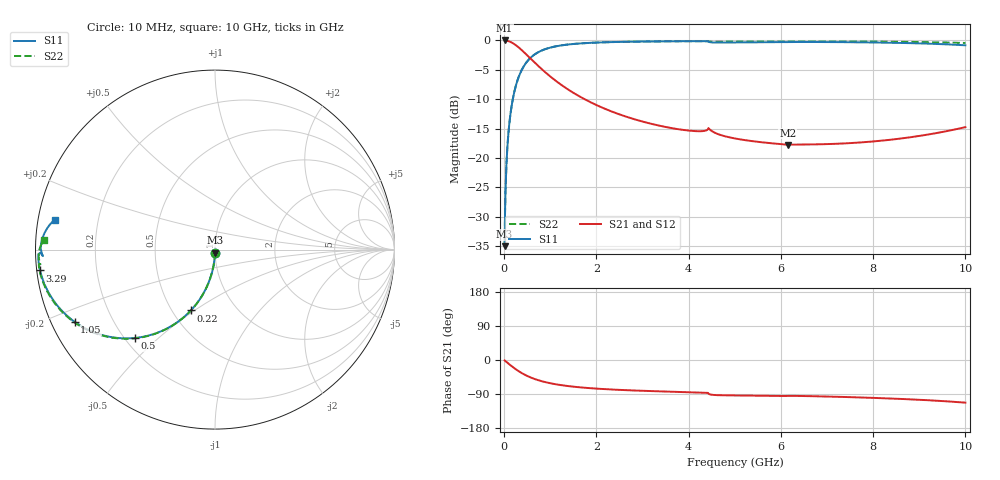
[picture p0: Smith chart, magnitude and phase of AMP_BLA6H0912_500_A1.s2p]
! Created Mon Feb  1 16:19:20 2010
# hz S ma R 50
! 2 Port Network Data from SP1.SP block
! freq  magS11  angS11  magS21  angS21  magS12  angS12  magS22  angS22
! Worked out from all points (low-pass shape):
!   1000 points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, 10 MHz to 10 GHz, reference 50 ohm
!   highest |S21| = 0.00 dB at 10 MHz (marker M1); lowest = -17.7 dB at 6.15 GHz (marker M2)
!   |S21| within 3 dB of the highest: start of sweep to 562.3 MHz
!   lowest |S11| = -35.0 dB at 10 MHz (marker M3), VSWR 1.04, Z = 49.9 - j1.78 ohm
!   |S11| at or under -10 dB: start of sweep to 187.2 MHz
!   |S22| runs from -35.0 to -0.1 dB; largest |S21 - S12| = 0
!   S11 on the Smith chart (normalised r, x): 10 MHz: 1.00, -0.04; 220 MHz: 0.62, -0.48; 500 MHz: 0.24, -0.42; 1.05 GHz: 0.07, -0.24; 3.29 GHz: 0.01, -0.06; 10 GHz: 0.05, +0.09
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1e7  0.01782 -91.0  0.9998 -1.0  0.9998 -1.0  0.01782 -91.0
4e7  0.07112 -94.1  0.9975 -4.1  0.9975 -4.1  0.07112 -94.1
7e7  0.1238 -97.2  0.9923 -7.2  0.9923 -7.2  0.1238 -97.2
1e8  0.1755 -100.2  0.9845 -10.2  0.9845 -10.2  0.1755 -100.2
1.5e8  0.2582 -105.1  0.9661 -15.1  0.9661 -15.1  0.2582 -105.1
2.2e8  0.3649 -111.6  0.9311 -21.6  0.9311 -21.6  0.3649 -111.6
3.4e8  0.5177 -121.6  0.8556 -31.5  0.8556 -31.5  0.5177 -121.4
5e8  0.6641 -132.2  0.7477 -42.1  0.7477 -42.1  0.6641 -132.0
7.5e8  0.7986 -143.8  0.6018 -53.7  0.6018 -53.7  0.7986 -143.5
1.05e9  0.8792 -152.7  0.4764 -62.5  0.4764 -62.5  0.8792 -152.3
1.33e9  0.9183 -158.2  0.3959 -67.9  0.3959 -67.9  0.9183 -157.6
1.68e9  0.9451 -162.9  0.3267 -72.5  0.3267 -72.5  0.9451 -162.2
2.43e9  0.9706 -169.0  0.2407 -78.5  0.2407 -78.5  0.9706 -167.9
3.29e9  0.9815 -173.2  0.1914 -82.4  0.1914 -82.4  0.9815 -171.7
3.34e9  0.9819 -173.4  0.1895 -82.6  0.1895 -82.6  0.9819 -171.8
4.07e9  0.9854 -176.2  0.1703 -85.1  0.1703 -85.1  0.9854 -174.0
4.45e9  0.9686 -178.6  0.1762 -90.2  0.1762 -90.2  0.9782 -175.3
5.01e9  0.9622 -178.1  0.1466 -93.5  0.1466 -93.5  0.9786 -175.6
6.15e9  0.9698 -179.9  0.1296 -94.6  0.1296 -94.6  0.9829 -177.2
6.67e9  0.9704 178.9  0.1306 -95.5  0.1306 -95.5  0.983 -178.1
8.34e9  0.9566 174.9  0.1427 -101.4  0.1427 -101.4  0.9761 179.5
1e10  0.909 169.5  0.1832 -112.6  0.1832 -112.6  0.9516 176.7
